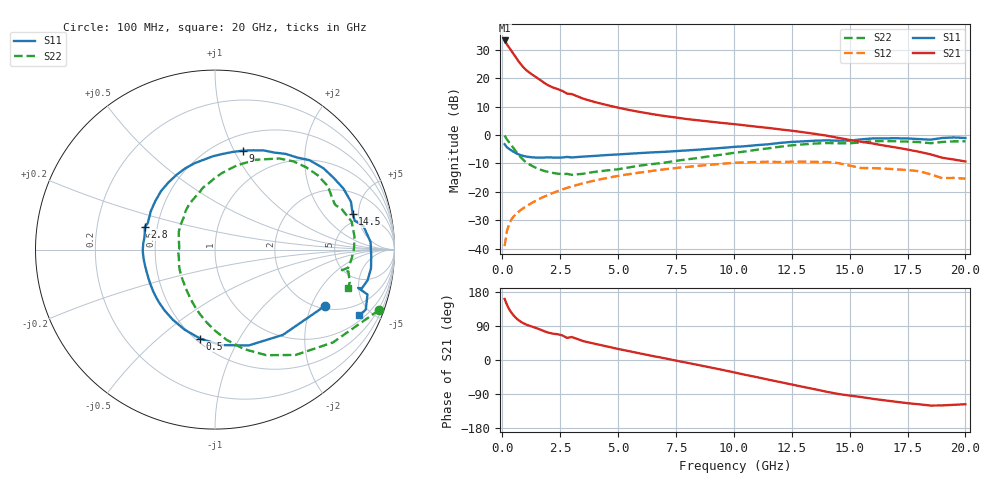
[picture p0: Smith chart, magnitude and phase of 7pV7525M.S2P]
! Infineon Technologies  Discrete & RF Semiconductors
! bfp620
! VCE = 0.75 V,  IC =  25 mA
! Common Emitter S-Parameters:  Sep 2002
# GHz  S  MA  R  50
!  f  S11  S21  S12  S22
! GHz  MAG  ANG  MAG  ANG  MAG  ANG  MAG  ANG
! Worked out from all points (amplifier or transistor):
!   59 points, 100 MHz to 20 GHz, reference 50 ohm
!   highest |S21| = 33.2 dB at 100 MHz (marker M1)
!   |S21| within 3 dB of that: start of sweep to 338.7 MHz
!   unconditionally stable (mu >= 1): 3.268 GHz to 10.13 GHz; 17.06 GHz to end of sweep
!   at 1 GHz: K = 0.75, MSG = 24.2 dB, |S12| = -25.3 dB
!   at 5.5 GHz: K = 1.04, MAG = 10.0 dB, |S12| = -13.7 dB
!   at 20 GHz: K = 1.45, MAG = -1.0 dB, |S12| = -15.4 dB
!   S11 on the Smith chart (normalised r, x): 100 MHz: 2.11, -2.52; 500 MHz: 0.53, -0.70; 2.8 GHz: 0.43, +0.13; 9 GHz: 0.66, +1.08; 14.5 GHz: 3.95, +4.24; 20 GHz: 1.26, -4.25
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0.1  0.6881 -27.2  45.81 161.2  0.0111 80.7  0.9745 -20.2
0.2  0.6072 -51.5  39.1 145.8  0.0204 67.7  0.8364 -38.2
0.3  0.566 -70.7  34.15 133.7  0.0275 62.2  0.7389 -52.6
0.4  0.5331 -86.3  29.88 124.3  0.0329 58.7  0.6539 -64.1
0.5  0.5028 -99.5  26.04 116.8  0.0374 56.3  0.5762 -73.9
0.6  0.4767 -111.0  22.66 110.5  0.0412 54.6  0.5072 -82.6
0.7  0.456 -121.0  19.81 105.3  0.0447 53.6  0.4492 -90.4
0.8  0.4403 -129.6  17.48 101.0  0.048 52.9  0.4025 -97.5
0.9  0.4288 -136.7  15.65 97.4  0.0513 52.6  0.3662 -103.7
1.1  0.4133 -147.6  13.12 91.9  0.0579 52.3  0.3164 -113.9
1.9  0.402 -177.1  7.814 74.0  0.0855 49.7  0.228 -149.1
2.8  0.4113 162.0  5.326 58.3  0.1174 43.7  0.2074 -179.4
3  0.4025 158.7  5.234 60.7  0.1245 42.1  0.1991 178.4
3.5  0.4167 149.2  4.339 49.7  0.142 37.7  0.208 165.4
5  0.4549 124.9  3.02 29.2  0.1908 23.4  0.2495 134.4
7  0.505 97.0  2.156 4.7  0.2486 3.6  0.3253 106.4
9  0.5724 74.4  1.71 -19.8  0.3 -17.7  0.4249 85.4
10.5  0.6348 58.3  1.472 -39.2  0.3306 -36.1  0.5135 70.5
13.5  0.7922 25.4  1.046 -77.2  0.3364 -71.3  0.7066 35.9
14.5  0.7925 14.6  0.891 -89.5  0.3206 -86.5  0.7133 24.0
17  0.8755 -6.9  0.602 -110.2  0.2492 -102.3  0.775 0.6
20  0.8847 -24.5  0.342 -116.8  0.1705 -113.2  0.7729 -16.2
